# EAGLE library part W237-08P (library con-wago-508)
WAGO SREW CLAMP
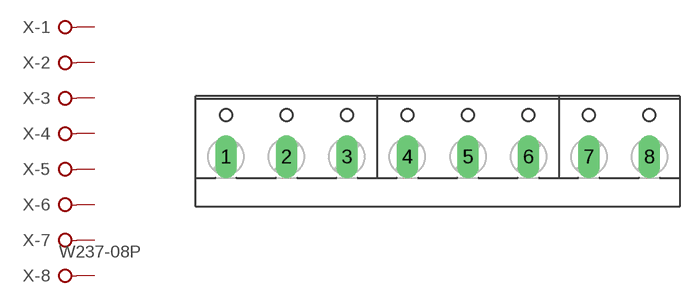
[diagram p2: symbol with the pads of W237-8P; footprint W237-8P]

Designator prefix X; gates -1=KL -2=KL -3=KL -4=KL -5=KL -6=KL -7=KL -8=KL+V

## W237-08P (OC_FARNELL: unknown; OC_NEWARK: unknown)  [W237-8P]
1  -1:KL  pas
2  -2:KL  pas
3  -3:KL  pas
4  -4:KL  pas
5  -5:KL  pas
6  -6:KL  pas
7  -7:KL  pas
8  -8:KL  pas

## Footprint W237-8P (pad centres in mm)
WAGO SREW CLAMP
drill 1.194 long: 1 -17.78,-0.635; 2 -12.7,-0.635; 3 -7.62,-0.635; 4 -2.54,-0.635; 5 2.54,-0.635; 6 7.62,-0.635; 7 12.7,-0.635; 8 17.78,-0.635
